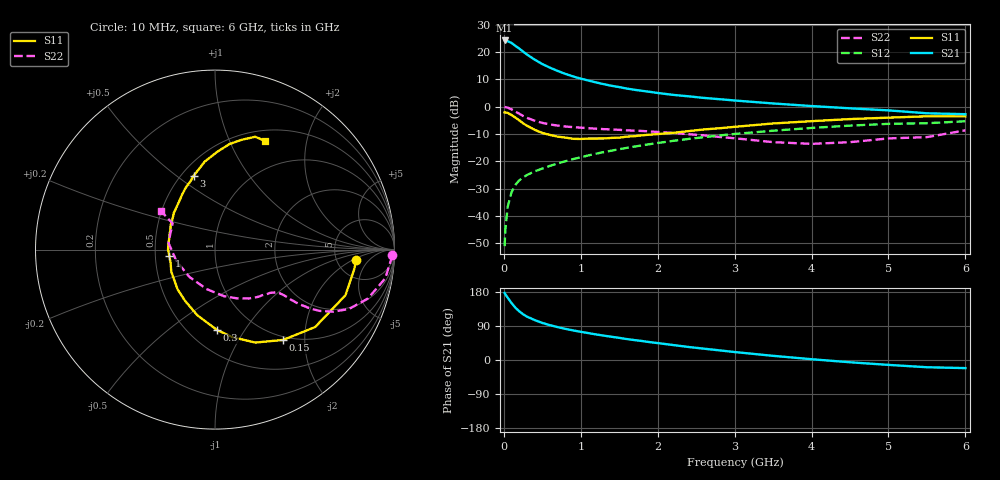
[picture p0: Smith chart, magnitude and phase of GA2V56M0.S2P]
! Infineon Technologies  Discrete & RF Semiconductors
! BF775
! Si NPN RF Bipolar Junction Transistor in SOT23
! VCE = 2.5 V  IC = 6 mA
! Common Emitter S-Parameters:  May  1996
# GHz  S  MA  R  50
!  f  S11  S21  S12  S22
! GHz  MAG  ANG  MAG  ANG  MAG  ANG  MAG  ANG
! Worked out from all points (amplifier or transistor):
!   36 points, 10 MHz to 6 GHz, reference 50 ohm
!   highest |S21| = 24.2 dB at 10 MHz (marker M1)
!   |S21| within 3 dB of that: start of sweep to 200.8 MHz
!   unconditionally stable (mu >= 1): 713.7 MHz to 3.629 GHz
!   at 250 MHz: K = 0.55, MSG = 23.0 dB, |S12| = -25.9 dB
!   at 1.4 GHz: K = 1.13, MAG = 9.7 dB, |S12| = -16.1 dB
!   at 6 GHz: K = 0.98, MSG = 1.3 dB, |S12| = -5.3 dB
!   S11 on the Smith chart (normalised r, x): 10 MHz: 7.70, -2.41; 150 MHz: 0.94, -1.58; 300 MHz: 0.68, -0.76; 1 GHz: 0.59, -0.04; 3 GHz: 0.57, +0.58; 6 GHz: 0.63, +1.37
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0.01  0.7887 -4.3  16.31 176.8  0.0028 87.7  0.9887 -1.9
0.02  0.7835 -7.9  16.11 173.3  0.0057 85.2  0.9801 -3.9
0.05  0.77 -19.3  15.79 164.4  0.0147 79.8  0.9618 -9.6
0.1  0.7053 -37.7  14.69 150.3  0.0273 72.3  0.8949 -17.7
0.15  0.6303 -53.0  13.01 138.0  0.0371 65.3  0.8166 -23.9
0.2  0.5644 -66.6  11.57 128.6  0.0448 61.6  0.744 -27.7
0.25  0.4969 -78.8  10.2 120.6  0.0507 58.7  0.6773 -30.3
0.3  0.4489 -88.4  9.029 114.5  0.0561 57.8  0.626 -31.7
0.4  0.3785 -105.2  7.276 105.5  0.0655 56.3  0.5542 -33.0
0.5  0.3303 -120.4  6.033 97.8  0.0737 56.8  0.5054 -33.4
0.6  0.3045 -133.1  5.172 91.9  0.0826 57.1  0.473 -33.4
0.7  0.2829 -143.7  4.51 86.7  0.0915 57.8  0.4509 -33.7
0.8  0.2724 -153.5  3.983 82.2  0.1005 58.2  0.4345 -34.0
1  0.2565 -172.1  3.264 74.4  0.1186 58.6  0.4133 -35.2
1.1  0.2615 179.9  3.007 70.9  0.1284 58.6  0.4041 -36.4
1.6  0.2833 150.8  2.146 55.2  0.1768 56.6  0.3693 -43.1
2.2  0.3318 127.5  1.647 39.5  0.2368 52.0  0.3317 -55.2
3  0.4281 106.1  1.299 21.0  0.3171 43.3  0.2644 -79.1
3.5  0.4932 96.7  1.146 11.0  0.3634 37.1  0.2245 -102.2
4.5  0.5935 82.2  0.934 -6.0  0.4506 23.9  0.2243 -163.5
5.5  0.6672 70.4  0.757 -19.1  0.4983 9.2  0.2775 148.2
6  0.6668 65.2  0.729 -21.4  0.5417 5.1  0.369 144.6
